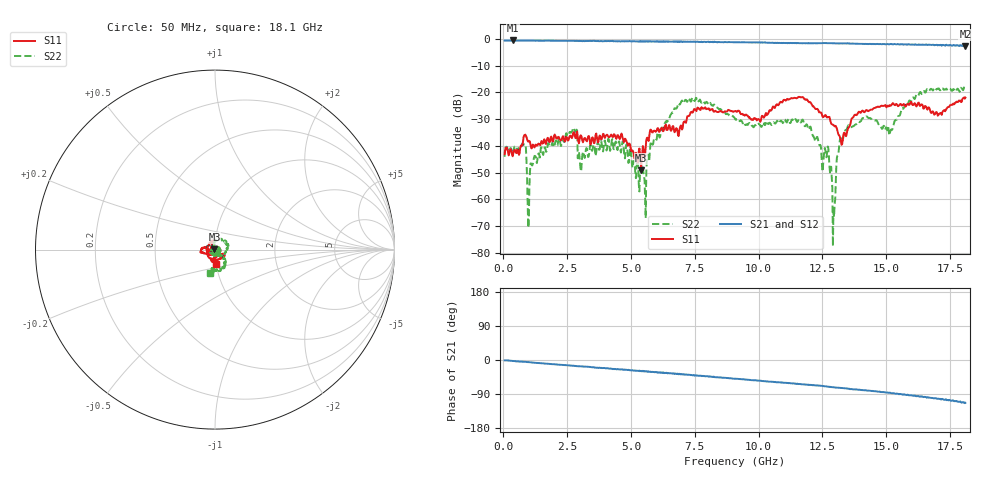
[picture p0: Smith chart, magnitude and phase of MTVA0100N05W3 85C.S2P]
! Network Analyzer HP8720D.06.14 Serial No. US36140669
! 17 Jan 2005  09:11:09
! Frequency  S11  S21  S12  S22
# HZ  S  DB R 50
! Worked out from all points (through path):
!   801 points, 50 MHz to 18.1 GHz, reference 50 ohm
!   highest |S21| = -0.59 dB at 365.9 MHz (marker M1); lowest = -2.8 dB at 18.1 GHz (marker M2)
!   group delay of S21, straight-line fit = 16.4 ps
!   lowest |S11| = -49.2 dB at 5.397 GHz (marker M3), VSWR 1.01, Z = 49.7 + j0.133 ohm
!   |S11| at or under -10 dB: start of sweep to end of sweep
!   |S22| runs from -77.5 to -17.6 dB; largest |S21 - S12| = 0.029
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5e7  -43.15 -26.5  -0.61 -0.9  -0.62 -1.1  -44.09 -5.9
3.65875e8  -43.90 2.2  -0.59 -2.7  -0.62 -2.7  -43.00 -4.9
7.945625e8  -36.66 34.4  -0.70 -4.7  -0.66 -4.9  -39.62 -22.5
1.020188e9  -38.20 2.5  -0.64 -5.8  -0.65 -6.2  -55.75 146.1
1.155562e9  -39.54 15.3  -0.66 -6.8  -0.65 -7.2  -46.83 88.6
2.689812e9  -37.10 37.1  -0.70 -14.9  -0.72 -15.3  -34.65 109.8
3.073375e9  -37.01 53.7  -0.80 -17.0  -0.76 -17.3  -45.73 -86.4
4.47225e9  -35.99 31.0  -0.93 -23.9  -0.88 -24.4  -41.59 132.4
5.397312e9  -49.22 157.3  -0.90 -28.5  -0.89 -28.9  -48.43 45.6
5.510125e9  -42.38 177.7  -0.97 -30.4  -0.99 -30.5  -51.03 177.2
6.074188e9  -33.70 -136.4  -1.05 -33.4  -1.03 -33.5  -35.44 128.4
7.202312e9  -29.01 119.4  -0.99 -38.7  -1.04 -39.3  -23.54 42.2
9.075e9  -27.05 -165.4  -1.27 -49.3  -1.26 -49.6  -29.81 -72.3
1.209838e10  -24.80 -157.2  -1.58 -66.3  -1.62 -66.5  -35.57 -174.8
1.266244e10  -29.19 -130.3  -1.56 -69.9  -1.59 -70.2  -44.28 -166.9
1.293319e10  -32.23 -129.6  -1.64 -72.1  -1.61 -72.4  -62.84 -114.8
1.313625e10  -35.95 -125.5  -1.73 -73.2  -1.72 -73.5  -42.02 -19.3
1.345212e10  -35.52 -131.3  -1.69 -74.8  -1.71 -75.2  -33.77 -54.2
1.509919e10  -25.21 -106.2  -2.05 -86.8  -1.93 -87.1  -34.74 -88.3
1.624988e10  -23.91 -31.7  -2.19 -95.0  -2.17 -95.8  -21.27 -53.1
1.708469e10  -27.93 -71.3  -2.36 -102.8  -2.20 -103.5  -18.97 -86.2
1.81e10  -21.99 -87.4  -2.78 -113.2  -2.64 -114.2  -17.65 -101.1
